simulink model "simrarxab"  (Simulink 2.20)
settings: Solver=VariableStepDiscrete  StartTime=0.0  StopTime=800  RelTol=1e-3  AbsTol=1e-6

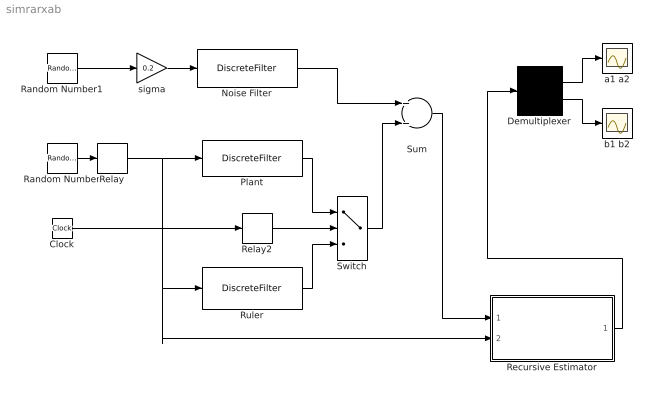
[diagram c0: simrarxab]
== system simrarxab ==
  Clock : Clock
  Demultiplexer : Demux  Outputs=2
  Noise Filter : DiscreteFilter  Numerator=[1 -1 0.2]  Denominator=[1 -1.5 0.7]  SampleTime=1
  Plant : DiscreteFilter  Numerator=[1 0.5]  Denominator=[1 -1.5 0.7]  SampleTime=1
  Random Number : RandomNumber  Mean=0  Variance=1  Seed=123456789  SampleTime=1
  Random Number1 : RandomNumber  Mean=0  Variance=1  Seed=123459  SampleTime=1
  Recursive Estimator : Subsystem  mask(Recursive Estimator){nn=[2 2 1], ff=0.98, pdiag=10000, ts=1}
      mask prompts: nn "ARX model structure [na nb nk]  :"; ff "Forgetting factor  ff :"; pdiag "Íà÷àëíà ñòîéíîñò çà äèàãîíàëà íà êîâàðèàöèîííàòà ìàòðèöà  P  :"; ts "How often to sample points [sec] :"
      mask help: Recursive parameter estimation
      mask init:
      | nn=@1; ff=@2; pdiag=@3; ts=@4;
      | na=nn(1); d=na+nn(2); dm=sum(nn)-1;
      | i=[1:na  na+nn(3):dm];  ii=[1:dm];
  Relay : Relay  OnSwitchValue=eps  OffSwitchValue=eps  OnOutputValue=-1  OffOutputValue=1
  Relay2 : Relay  OnSwitchValue=200  OffSwitchValue=200  OnOutputValue=-1  OffOutputValue=1
  Ruler : DiscreteFilter  Numerator="[0.5  -0.25]"  Denominator="[1 1.5  0.7]"  SampleTime=1
  Sum : Sum  Inputs=++
  Switch : Switch  Threshold=0
  a1 a2 : Scope
  b1 b2 : Scope
  sigma : Gain  Gain=0.2
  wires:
  Random Number/1 -> Relay/1
  Random Number1/1 -> sigma/1
  sigma/1 -> Noise Filter/1
  Noise Filter/1 -> Sum/1
  Relay/1 -> Plant/1, Recursive Estimator/2(u (k)), Ruler/1
  Ruler/1 -> Switch/3
  Plant/1 -> Switch/1
  Switch/1 -> Sum/2
  Relay2/1 -> Switch/2
  Clock/1 -> Relay2/1
  Sum/1 -> Recursive Estimator/1(y (k))
  Demultiplexer/2 -> b1 b2/1
  Demultiplexer/1 -> a1 a2/1
  Recursive Estimator/1(tetha (k)) -> Demultiplexer/1

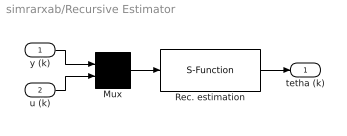
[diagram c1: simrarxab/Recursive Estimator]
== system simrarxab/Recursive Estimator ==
  y (k) : Inport  Port=1  PortWidth=-1  SampleTime=-1
  u (k) : Inport  Port=2  PortWidth=-1  SampleTime=-1
  Mux : Mux  Inputs=2
  Rec. estimation : S-Function  FunctionName=rarxm_sl  Parameters=na,ff,pdiag,ts,d,dm,i,ii  PortCounts=[]  SFunctionModules=''
  tetha (k) : Outport  Port=1
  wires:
  Rec. estimation/1 -> tetha (k)/1
  Mux/1 -> Rec. estimation/1
  u (k)/1 -> Mux/2
  y (k)/1 -> Mux/1
